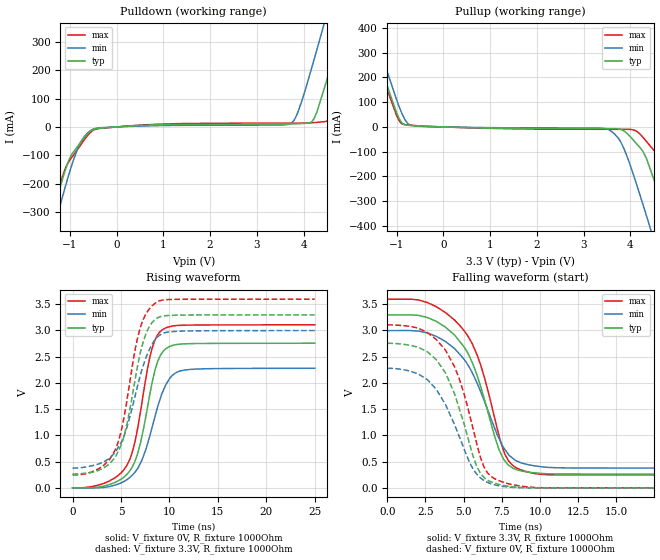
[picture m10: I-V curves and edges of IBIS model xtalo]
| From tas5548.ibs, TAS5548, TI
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|   xtalo Model
[Model]   xtalo
Model_type   Output
Polarity   Non-Inverting
Vmeas = 1.65
Vref = 0
Cref = 1pF
Rref = 1000000
|   typ   min   max
C_comp   1.334pF   1.322pF   1.371pF
[Voltage Range]   3.3   3   3.6
[Temperature Range]   27   125   0
[Pullup Reference]   3.3   3   3.6
[Pulldown Reference]   -0   -0   -0
[Power Clamp Reference]   3.3   3   3.6
[GND Clamp Reference]   -0   -0   -0
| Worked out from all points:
|   slope of the pulldown table from 0 to 0.495 V, typ, clamps not added: 96.4 ohm
|   slope of the pullup table from 0 to 0.495 V, typ, clamps not added: 194 ohm
|   falling waveform, V_fixture 3.3V, R_fixture 1000Ohm: 20-80 % time 2.14ns typ, 2.42ns min, 2.19ns max; typ from 3.3 V to 0.263 V
|   rising waveform, V_fixture 0V, R_fixture 1000Ohm: 20-80 % time 1.93ns typ, 2.32ns min, 1.91ns max; typ from 0.002 V to 2.76 V
|   rising waveform, V_fixture 3.3V, R_fixture 1000Ohm: 20-80 % time 2.04ns typ, 2.45ns min, 2.03ns max; typ from 0.263 V to 3.3 V
|   falling waveform, V_fixture 0V, R_fixture 1000Ohm: 20-80 % time 1.9ns typ, 2.11ns min, 1.99ns max; typ from 2.76 V to 0.002 V
[Pulldown]
|   Voltage   I(typ)   I(min)   I(max)
-3.3V     -1.528A    -1.578A    -1.516A
-1.934V   -661.2mA   -722.3mA   -646mA
-1.34V    -291.4mA   -356.8mA   -276.1mA
-1.082V   -145.3mA   -203.2mA   -141.5mA
-825mV    -66.98mA   -72.85mA   -77.58mA
-468.6mV  -7.265mA   -5.934mA   -9.27mA
3.729V    10.6mA     12mA       13.46mA
4.184V    19.87mA    213.7mA    14.82mA
4.481V    155.5mA    387.4mA    19.29mA
4.877V    392.8mA    625.1mA    198.9mA
5.194V    587.8mA    815.3mA    391.2mA
6.58V     1.442A     1.648A     1.253A
[Pullup]
|   Voltage   I(typ)   I(min)   I(max)
-3.3V     1.454A     1.479A     1.451A
-1.617V   416.7mA    468.4mA    404.7mA
-884.4mV  15.62mA    52.75mA    12.42mA
-547.8mV  3.903mA    2.808mA    4.769mA
3.472V    -7.102mA   -6.894mA   -9.581mA
3.769V    -8.757mA   -53.3mA    -9.665mA
4.066V    -53.71mA   -193.4mA   -11.95mA
4.343V    -126.5mA   -358.5mA   -58.43mA
4.818V    -401mA     -650.3mA   -205.8mA
5.095V    -574mA     -822.6mA   -370.9mA
5.234V    -661.1mA   -908.8mA   -457.3mA
6.58V     -1.516A    -1.754A    -1.311A
[Ramp]
R_load = 1000
|   typ   min   max
dV/dt_r   1.65253/1.93115e-09   1.36637/2.32255e-09   1.86273/1.91372e-09
dV/dt_f   1.81981/2.13902e-09   1.57234/2.4212e-09   2.00925/2.18933e-09
[Falling Waveform]
V_fixture = 3.3V
V_fixture_min = 3V
V_fixture_max = 3.6V
R_fixture = 1000Ohm
C_fixture = 0F
|   Time   V(typ)   V(min)   V(max)
0s        3.296V     2.997V     3.596V
2.624ns   3.247V     2.953V     3.532V
3.812ns   3.062V     2.79V      3.341V
5.016ns   2.69V      2.455V     3V
6.113ns   1.932V     1.833V     2.341V
7.308ns   733.6mV    948mV      1.006V
7.703ns   514.9mV    732.5mV    640mV
8.469ns   348.9mV    514.9mV    380.1mV
10.51ns   269.6mV    392.1mV    252.2mV
25ns      263.4mV    376.2mV    247.1mV
[Rising Waveform]
V_fixture = 0V
V_fixture_min = 0V
V_fixture_max = 0V
R_fixture = 1000Ohm
C_fixture = 0F
|   Time   V(typ)   V(min)   V(max)
0s        1.625mV    1.647mV    1.851mV
3.218ns   32.83mV    8.14mV     85.84mV
5.555ns   248.6mV    150.2mV    413.2mV
6.113ns   381.1mV    233.1mV    649mV
6.709ns   647.4mV    367.6mV    1.129V
8.213ns   2.009V     1.155V     2.66V
9.319ns   2.593V     1.835V     3.02V
10.26ns   2.711V     2.136V     3.082V
11.54ns   2.744V     2.245V     3.1V
25ns      2.756V     2.279V     3.106V
[Rising Waveform]
V_fixture = 3.3V
V_fixture_min = 3V
V_fixture_max = 3.6V
R_fixture = 1000Ohm
C_fixture = 0F
|   Time   V(typ)   V(min)   V(max)
0s        263.4mV    376.2mV    247.1mV
2.624ns   329.3mV    451.6mV    357.6mV
4.406ns   581.7mV    675.6mV    722.6mV
5.382ns   1.035V     1.029V     1.416V
6.329ns   1.929V     1.656V     2.503V
6.976ns   2.558V     2.131V     3.045V
7.607ns   2.953V     2.498V     3.322V
8.469ns   3.2V       2.81V      3.51V
10.51ns   3.289V     2.98V      3.59V
25ns      3.296V     2.997V     3.596V
[Falling Waveform]
|Gnd
V_fixture = 0V
V_fixture_min = 0V
V_fixture_max = 0V
R_fixture = 1000Ohm
C_fixture = 0F
|   Time   V(typ)   V(min)   V(max)
0s        2.756V     2.279V     3.106V
2.03ns    2.68V      2.171V     3.043V
3.218ns   2.44V      1.875V     2.824V
3.812ns   2.191V     1.587V     2.623V
4.703ns   1.518V     984.7mV    2.086V
5.868ns   402.8mV    259.7mV    827.5mV
6.329ns   203mV      139.9mV    401.3mV
7.192ns   77.24mV    48.34mV    153mV
10ns      3.001mV    3.807mV    4.454mV
25ns      1.627mV    1.68mV     1.85mV
